|   IBIS model for TI TMS320TCI6457 DSP
[IBIS Ver]   5.0
[Disclaimer]   Please be aware that in the absence of a written agreement
|   Texas Instruments(TI) assumes no liability for:
|   (1) The accuracy of the IBIS models provided to your company
|   (2) The proper functioning of these Models in your design
|   or for any resulting applications
|   (3) Infringement of patents, copyrights or intellectual
|   property rights resulting from your use of these
|   models.
|   TI provides IBIS Models as a service to our customers and
|   therefore reserves the right to limit distribution of the
|   Models.  The information is subject to change without notice.
[File Name]  tms320c6457c.ibs
[File Rev]   1.2
[Date]   March 30, 2011
[Source]   File Originated at Texas Instruments
|   Revision 1.2 -- 30 March 2011 - [R. Lerner]
|   -Updated bshtltcscdvgpbfz ibis model
|   -IBISCHK5 resulted in 0 errors and 37 warnings (listed below)
|   Revision 1.1 -- 2/14/2011
|   cleaned uprevision history
|   -108 Warnings identified
|   Revision 1.0 -- 5/26/2010 [Initial full release]
|   Updated IO buffer models added
|   -BC1840DTHYPDFZ
|   -BC1840ETHYFZ
|   -ICLKRX18G
|   -IC18THYPUFZ
|   -IC18THYPDFZ
|   -IC18THY
|   -IC18GHY
|   -BSHTLTCSCDVGPBFZ
|   the following portions of the model have been updated
|   Driver:
|   a) Impedance   - 45/50/55 ohms impedance
|   b) Slew Rate Operation   - Fast and slow modes of operation
|   c) Voltage Levels   - 1.5/1.8V
|   d) Voltage Nom variation   - 10%/5%
|   Reciever -
|   a) Termination Modes  - Half/Full Termination as well as no termination modes
|   b) Termination Impedance   - 45/50/55 ohms impedance
|   c) Voltage Levels   - 1.5/1.8V
|   d) Voltage Nom variation   - 10%/5%
|   -BI2C18TFZ
|   -BC1850CTHYPUFZ
|   -BC1840ETHYPDFZ
|   -BC1825ETHYPUFZ
|   -BC1825ETHYPDFZ
|   -BQ3350ZTCBTHYPBFZP18
|   -BQ3340ZTCDTHYPBFZP18
|   -BC1850CTHYPDFZ
|   Note: Updated BC1825ETHYPUFZ model missing
|   IBIS Checker updated
|   IBIS Quality Notes added
|   File passes ibischk5.0.3 with 0 errors and 4 warnings.
|   Revision 0.3 -- 1/29/2009
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[Copyright]   Property of Texas Instruments Incorporated.
|   Unauthorized reproduction and/or distribution is strictly
|   prohibited.
|   This product is protected under copyright law and trade
|   secret law as an unpublished work.
|   Created 2008,(C) Copyright 1999-2011,
|   Texas Instruments Incorporated., All Rights Reserved.
|   These commodities are under the U.S.
|   Government distribution license control.As such,they are not
|   to be re-exported without the prior approval of the U.S.
|   Department of Commerce.
[Notes]
|   Some IV curves contain Non monotonic data points.
|   Some reserved pins (RSVxx) are listed as NC, these pins may
|   require either a pull up or pull down resistor to the
|   appropriate rail - refer to your data manual for proper connection
|   IBIS Quality Notes
|   Component TMS320TCI6457: Over all Quality Level 2A
|  IQ
|  IQ  IBISCHK5 V5.0.4
|  IQ
|  IQ  Buffer Model BC1840DTHYPDFZ: IQ Level 2A
|  IQ   -Warning: POWER Clamp, Typical value never becomes zero
|  IQ   -Warning: POWER Clamp, Minimum value never becomes zero
|  IQ   -Warning: POWER Clamp, Maximum value never becomes zero
|  IQ   -Note: Pull down/up min/typ/max data is non-monotonic
|  IQ  Buffer Model ICLKRX18G: IQ Level 2A
|  IQ   -Warning: POWER Clamp, Typical value never becomes zero
|  IQ   -Warning: POWER Clamp, Minimum value never becomes zero
|  IQ   -Warning: POWER Clamp, Maximum value never becomes zero
|  IQ   -Note: Pull down/up min/typ/max data is non-monotonic
|  IQ  Buffer Model IC18THYPUFZ: IQ Level 2A
|  IQ   -Warning: GND Clamp, Typical value never becomes zero
|  IQ   -Warning: GND Clamp, Maximum value never becomes zero
|  IQ   -Note: Pull down/up min/typ/max data is non-monotonic
|  IQ  Buffer Model IC18THYPDFZ: IQ Level 2A
|  IQ   -Warning: POWER Clamp, Typical value never becomes zero
|  IQ   -Warning: POWER Clamp, Minimum value never becomes zero
|  IQ   -Warning: POWER Clamp, Maximum value never becomes zero
|  IQ  Buffer Model BC1850CTHYPUFZ: IQ Level 2A
|  IQ   -Warning: GND Clamp, Typical value never becomes zero
|  IQ   -Warning: GND Clamp, Maximum value never becomes zero
|  IQ   -Note: Pull down/up min/typ/max data is non-monotonic
|  IQ  Buffer Model BC1840ETHYPDFZ: IQ Level 2A
|  IQ   -Warning: POWER Clamp, Typical value never becomes zero
|  IQ   -Warning: POWER Clamp, Minimum value never becomes zero
|  IQ   -Warning: POWER Clamp, Maximum value never becomes zero
|  IQ   -Note: Pull down/up min/typ/max data is non-monotonic
|  IQ  Buffer Model BC1825ETHYPUFZ: IQ Level 2A
|  IQ   -Warning: GND Clamp, Typical value never becomes zero
|  IQ   -Warning: GND Clamp, Maximum value never becomes zero
|  IQ   -Note: Pull down/up min/typ/max data is non-monotonic
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[Component] TMS320C6457
[Manufacturer] Texas Instruments
[Package Model] 6457
[Package]
||Variable   Typ   Min   Max
R_pkg   1.77   0.845   3.51
L_pkg   3.61nH  2.22nH   6.22nH
C_pkg   1.76pF  1.22pF   2.84pF
[Pin]   signal_name   model_name
G6   DDRCLKSEL   IC18GHY
AE19   NMI   BC1850CTHYPDFZ
AF6   ALTCORECLK   IC18THY
AF23   RESETSTATZ   BC1850CTHYPDFZ
AH6   CORECLKP   ICLKRX18G
AH23   RESETZ   IC18THY
AD7   SYSCLKOUT   BC1840ETHYPDFZ
AG22   PORZ   IC18THY
AG7   RIOSGMIICLKP   ICLKRX18G
AG6   RIOSGMIICLKN   ICLKRX18G
AE6   CORECLKSEL   IC18GHY
E6   DDRREFCLKN   ICLKRX18G
D6   DDRREFCLKP   ICLKRX18G
AH7   CORECLKN   ICLKRX18G
C6   ALTDDRCLK   IC18THY
E22   DDRDQS3P   BSHTLTCSCDVGPBFZ
B6   DDRD14   BSHTLTCSCDVGPBFZ
E8   DDRD10   BSHTLTCSCDVGPBFZ
A15   DDRA11   BSHTLTCSCDVGPBFZ
C8   DDRD08   BSHTLTCSCDVGPBFZ
D21   DDRD27   BSHTLTCSCDVGPBFZ
D18   DDRD19   BSHTLTCSCDVGPBFZ
A24   DDRD30   BSHTLTCSCDVGPBFZ
C12   DDRWEZ   BSHTLTCSCDVGPBFZ
C19   DDRDQM2   BSHTLTCSCDVGPBFZ
A27   DDRSLRATE   BC1840ETHYFZ
A21   DDRD24   BSHTLTCSCDVGPBFZ
D11   DDRD03   BSHTLTCSCDVGPBFZ
D7   DDRDQS1N   BSHTLTCSCDVGPBFZ
F17   DDRA00   BSHTLTCSCDVGPBFZ
B21   DDRD25   BSHTLTCSCDVGPBFZ
B17   DDRCLKOUTN1   BSHTLTCSCDVGPBFZ
E17   DDRA01   BSHTLTCSCDVGPBFZ
C16   DDRA06   BSHTLTCSCDVGPBFZ
C22   DDRDQM3   BSHTLTCSCDVGPBFZ
A20   DDRD20   BSHTLTCSCDVGPBFZ
B15   DDRA10   BSHTLTCSCDVGPBFZ
E13   DDRCEZ   BSHTLTCSCDVGPBFZ
C11   DDRD02   BSHTLTCSCDVGPBFZ
C17   DDRA03   BSHTLTCSCDVGPBFZ
D20   DDRD23   BSHTLTCSCDVGPBFZ
D8   DDRD09   BSHTLTCSCDVGPBFZ
D19   DDRDQS2N   BSHTLTCSCDVGPBFZ
A10   DDRD04   BSHTLTCSCDVGPBFZ
C15   DDRA09   BSHTLTCSCDVGPBFZ
D16   DDRA05   BSHTLTCSCDVGPBFZ
B16   DDRA07   BSHTLTCSCDVGPBFZ
E10   DDRDQS0P   BSHTLTCSCDVGPBFZ
B12   DDRD01   BSHTLTCSCDVGPBFZ
B9   DDRRCVENOUT0   BSHTLTCSCDVGPBFZ
F20   DDRRCVENOUT1   BSHTLTCSCDVGPBFZ
D12   DDRRASZ   BSHTLTCSCDVGPBFZ
E16   DDRA04   BSHTLTCSCDVGPBFZ
E15   DDRODT   BSHTLTCSCDVGPBFZ
C18   DDRD18   BSHTLTCSCDVGPBFZ
D13   DDRCKE   BSHTLTCSCDVGPBFZ
A18   DDRD17   BSHTLTCSCDVGPBFZ
E7   DDRDQS1P   BSHTLTCSCDVGPBFZ
B10   DDRD05   BSHTLTCSCDVGPBFZ
B14   DDRA13   BSHTLTCSCDVGPBFZ
D14   DDRBA1   BSHTLTCSCDVGPBFZ
A14   DDRA12   BSHTLTCSCDVGPBFZ
B23   DDRD29   BSHTLTCSCDVGPBFZ
E19   DDRDQS2P   BSHTLTCSCDVGPBFZ
E20   DDRRCVENIN1   BSHTLTCSCDVGPBFZ
E12   DDRCASZ   BSHTLTCSCDVGPBFZ
B20   DDRD21   BSHTLTCSCDVGPBFZ
B13   DDRCLKOUTN0   BSHTLTCSCDVGPBFZ
A6   DDRD15   BSHTLTCSCDVGPBFZ
C7   DDRDQM1   BSHTLTCSCDVGPBFZ
A9   DDRRCVENIN0   BSHTLTCSCDVGPBFZ
C21   DDRD26   BSHTLTCSCDVGPBFZ
D17   DDRA02   BSHTLTCSCDVGPBFZ
F8   DDRD11   BSHTLTCSCDVGPBFZ
A17   DDRCLKOUTP1   BSHTLTCSCDVGPBFZ
B18   DDRD16   BSHTLTCSCDVGPBFZ
D15   DDRA08   BSHTLTCSCDVGPBFZ
E14   DDRBA2   BSHTLTCSCDVGPBFZ
B24   DDRD31   BSHTLTCSCDVGPBFZ
A23   DDRD28   BSHTLTCSCDVGPBFZ
D22   DDRDQS3N   BSHTLTCSCDVGPBFZ
B7   DDRD12   BSHTLTCSCDVGPBFZ
A13   DDRCLKOUTP0   BSHTLTCSCDVGPBFZ
D10   DDRDQS0N   BSHTLTCSCDVGPBFZ
D9   DDRD07   BSHTLTCSCDVGPBFZ
C10   DDRDQM0   BSHTLTCSCDVGPBFZ
C20   DDRD22   BSHTLTCSCDVGPBFZ
C9   DDRD06   BSHTLTCSCDVGPBFZ
C14   DDRBA0   BSHTLTCSCDVGPBFZ
A7   DDRD13   BSHTLTCSCDVGPBFZ
A12   DDRD00   BSHTLTCSCDVGPBFZ
P25   AEA16   BQ3350ZTCBTHYPBFZP18
AD26   AED12   BQ3350ZTCBTHYPBFZP18
AF24   AED03   BQ3350ZTCBTHYPBFZP18
N26   AEA07   BQ3350ZTCBTHYPBFZP18
U25   AEA00   BQ3350ZTCBTHYPBFZP18
V25   ABA0   BQ3350ZTCBTHYPBFZP18
F27   AED52   BQ3350ZTCBTHYPBFZP18
T25   AEA11   BQ3350ZTCBTHYPBFZP18
G26   AED50   BQ3350ZTCBTHYPBFZP18
AB25   AED26   BQ3350ZTCBTHYPBFZP18
H26   AED43   BQ3350ZTCBTHYPBFZP18
Y27   AED27   BQ3350ZTCBTHYPBFZP18
AC24   AED00   BQ3350ZTCBTHYPBFZP18
C28   AED41   BQ3350ZTCBTHYPBFZP18
J24   AED47   BQ3350ZTCBTHYPBFZP18
R26   AEA13   BQ3350ZTCBTHYPBFZP18
G27   AED48   BQ3350ZTCBTHYPBFZP18
AF28   AED30   BQ3350ZTCBTHYPBFZP18
B27   AED51   BQ3350ZTCBTHYPBFZP18
W27   ABE02Z   BQ3350ZTCBTHYPBFZP18
D25   AED57   BQ3350ZTCBTHYPBFZP18
D28   AED39   BQ3350ZTCBTHYPBFZP18
K25   AED46   BQ3350ZTCBTHYPBFZP18
AA24   ASDWEZ   BQ3350ZTCBTHYPBFZP18
L24   AED33   BQ3350ZTCBTHYPBFZP18
AE28   AED19   BQ3350ZTCBTHYPBFZP18
U28   AEA05   BQ3350ZTCBTHYPBFZP18
AE25   AOE   BQ3350ZTCBTHYPBFZP18
AG25   AED14   BQ3350ZTCBTHYPBFZP18
AB26   AED28   BQ3350ZTCBTHYPBFZP18
AA27   AED22   BQ3350ZTCBTHYPBFZP18
AF25   AED09   BQ3350ZTCBTHYPBFZP18
V26   ACE5Z   BQ3350ZTCBTHYPBFZP18
G25   AED36   BQ3350ZTCBTHYPBFZP18
R25   AADS   BQ3350ZTCBTHYPBFZP18
Y24   ABE01Z   BQ3350ZTCBTHYPBFZP18
AA25   AED23   BQ3350ZTCBTHYPBFZP18
T26   AEA02   BQ3350ZTCBTHYPBFZP18
N25   AHOLDAZ   BQ3350ZTCBTHYPBFZP18
J25   AED45   BQ3350ZTCBTHYPBFZP18
AC25   AED11   BQ3350ZTCBTHYPBFZP18
AB24   AED24   BQ3350ZTCBTHYPBFZP18
M26   AEA09   BQ3350ZTCBTHYPBFZP18
Y28   ABE03Z   BQ3350ZTCBTHYPBFZP18
G28   AED35   BQ3350ZTCBTHYPBFZP18
AE24   AED01   BQ3350ZTCBTHYPBFZP18
K28   AARDY   BQ3350ZTCBTHYPBFZP18
L28   ABE05Z   BQ3350ZTCBTHYPBFZP18
M24   AEA17   BQ3350ZTCBTHYPBFZP18
AC26   AED08   BQ3350ZTCBTHYPBFZP18
D27   AED58   BQ3350ZTCBTHYPBFZP18
W26   ACE2Z   BQ3350ZTCBTHYPBFZP18
AA28   AED29   BQ3350ZTCBTHYPBFZP18
N24   AEA10   BQ3350ZTCBTHYPBFZP18
E26   AED59   BQ3350ZTCBTHYPBFZP18
AE27   AED15   BQ3350ZTCBTHYPBFZP18
AF27   AED18   BQ3350ZTCBTHYPBFZP18
V24   ABA1   BQ3350ZTCBTHYPBFZP18
B26   AED49   BQ3350ZTCBTHYPBFZP18
C26   AED61   BQ3350ZTCBTHYPBFZP18
T28   AEA06   BQ3350ZTCBTHYPBFZP18
H24   AED55   BQ3350ZTCBTHYPBFZP18
AG27   AED20   BQ3350ZTCBTHYPBFZP18
U27   ACE4Z   BQ3350ZTCBTHYPBFZP18
J28   AED40   BQ3350ZTCBTHYPBFZP18
AC27   AED13   BQ3350ZTCBTHYPBFZP18
W28   ABE07Z   BQ3350ZTCBTHYPBFZP18
D26   AED53   BQ3350ZTCBTHYPBFZP18
T27   AEA03   BQ3350ZTCBTHYPBFZP18
AD27   AED04   BQ3350ZTCBTHYPBFZP18
AH26   AED06   BQ3350ZTCBTHYPBFZP18
N28   AECLKIN   BQ3350ZTCBTHYPBFZP18
Y25   ABE00Z   BQ3350ZTCBTHYPBFZP18
J26   AED44   BQ3350ZTCBTHYPBFZP18
A26   AED62   BQ3350ZTCBTHYPBFZP18
C27   AED60   BQ3350ZTCBTHYPBFZP18
H25   AED54   BQ3350ZTCBTHYPBFZP18
AF26   AED16   BQ3350ZTCBTHYPBFZP18
M25   AEA18   BQ3350ZTCBTHYPBFZP18
L27   ABE04Z   BQ3350ZTCBTHYPBFZP18
AE26   AED10   BQ3350ZTCBTHYPBFZP18
G24   AED63   BQ3350ZTCBTHYPBFZP18
K27   AED34   BQ3350ZTCBTHYPBFZP18
L26   ABUSREQ0   BQ3350ZTCBTHYPBFZP18
K24   AED38   BQ3350ZTCBTHYPBFZP18
U26   AEA01   BQ3350ZTCBTHYPBFZP18
Y26   AED31   BQ3350ZTCBTHYPBFZP18
W25   ACE3Z   BQ3350ZTCBTHYPBFZP18
P24   AEA19   BQ3350ZTCBTHYPBFZP18
AD28   AED17   BQ3350ZTCBTHYPBFZP18
F26   AED56   BQ3350ZTCBTHYPBFZP18
W24   ARNW   BQ3350ZTCBTHYPBFZP18
T24   AEA14   BQ3350ZTCBTHYPBFZP18
R24   AEA08   BQ3350ZTCBTHYPBFZP18
R27   AEA04   BQ3350ZTCBTHYPBFZP18
F28   AED37   BQ3350ZTCBTHYPBFZP18
P26   AEA15   BQ3350ZTCBTHYPBFZP18
J27   AED42   BQ3350ZTCBTHYPBFZP18
K26   AED32   BQ3350ZTCBTHYPBFZP18
N27   AEA12   BQ3350ZTCBTHYPBFZP18
AG26   AED02   BQ3350ZTCBTHYPBFZP18
AH25   AED05   BQ3350ZTCBTHYPBFZP18
AC28   AED21   BQ3350ZTCBTHYPBFZP18
V28   AECLKOUT   BQ3340ZTCDTHYPBFZP18
L25   ABE06Z   BQ3350ZTCBTHYPBFZP18
R28   AHOLDZ   BQ3350ZTCBTHYPBFZP18
AA26   AED25   BQ3350ZTCBTHYPBFZP18
AD25   AED07   BQ3350ZTCBTHYPBFZP18
AE4   EMU03   BC1825ETHYPUFZ
AH5   EMU02   BC1825ETHYPUFZ
AD5   EMU00   BC1825ETHYPUFZ
AD1   EMU15   BC1825ETHYPUFZ
AE3   EMU10   BC1825ETHYPUFZ
AG4   EMU05   BC1825ETHYPUFZ
AF2   EMU11   BC1825ETHYPUFZ
Y2   TMS   IC18THYPUFZ
AA1   EMU17   BC1825ETHYPUFZ
AE1   EMU12   BC1825ETHYPUFZ
AG2   EMU07   BC1825ETHYPUFZ
AB1   TDI   IC18THYPUFZ
AF3   EMU13   BC1825ETHYPUFZ
AF4   EMU06   BC1825ETHYPUFZ
AC1   EMU14   BC1825ETHYPUFZ
AD3   EMU16   BC1825ETHYPUFZ
AH3   TCK   IC18THYPUFZ
AC2   EMU18   BC1825ETHYPUFZ
AE5   EMU01   BC1825ETHYPUFZ
AH4   EMU04   BC1825ETHYPUFZ
AE2   TRSTZ   IC18THYPDFZ
AG3   EMU08   BC1825ETHYPUFZ
AF1   TDO   BC1840ETHYFZ
AD4   EMU09   BC1825ETHYPUFZ
D24   GP12   BC1825ETHYPDFZ
B25   GP08   BC1825ETHYPDFZ
C5   GP06   BC1825ETHYPDFZ
B5   GP04   BC1825ETHYPDFZ
F5   GP07   BC1825ETHYPDFZ
C25   GP11   BC1825ETHYPDFZ
B4   GP03   BC1825ETHYPDFZ
D5   GP02   BC1825ETHYPDFZ
A5   GP00   BC1825ETHYPUFZ
E5   GP01   BC1825ETHYPDFZ
A25   GP10   BC1825ETHYPDFZ
F6   GP05   BC1825ETHYPDFZ
C24   GP09   BC1825ETHYPDFZ
D23   GP14   BC1825ETHYPDFZ
F23   GP15   BC1825ETHYPDFZ
C23   GP13   BC1825ETHYPDFZ
R1   HD17   BQ3350ZTCBTHYPBFZP18
W1   HD11   BQ3350ZTCBTHYPBFZP18
P3   HD31   BQ3350ZTCBTHYPBFZP18
V1   HD22   BQ3350ZTCBTHYPBFZP18
T3   HD09   BQ3350ZTCBTHYPBFZP18
L2   HDS1Z   BQ3350ZTCBTHYPBFZP18
M1   HD24   BQ3350ZTCBTHYPBFZP18
W2   HD00   BQ3350ZTCBTHYPBFZP18
L6   HCNTL0   BQ3350ZTCBTHYPBFZP18
N4   HD12   BQ3350ZTCBTHYPBFZP18
U4   HD05   BQ3350ZTCBTHYPBFZP18
R6   HD04   BQ3350ZTCBTHYPBFZP18
N3   HD16   BQ3350ZTCBTHYPBFZP18
N5   HD08   BQ3350ZTCBTHYPBFZP18
R5   HD10   BQ3350ZTCBTHYPBFZP18
P4   HD14   BQ3350ZTCBTHYPBFZP18
U5   HD27   BQ3350ZTCBTHYPBFZP18
M6   HRDYZ   BQ3350ZTCBTHYPBFZP18
N1   HD26   BQ3350ZTCBTHYPBFZP18
K5   HRWZ   BQ3350ZTCBTHYPBFZP18
L3   HHWIL   BQ3350ZTCBTHYPBFZP18
N2   HD20   BQ3350ZTCBTHYPBFZP18
U1   HD21   BQ3350ZTCBTHYPBFZP18
T1   HD19   BQ3350ZTCBTHYPBFZP18
P5   HD02   BQ3350ZTCBTHYPBFZP18
T2   HD15   BQ3350ZTCBTHYPBFZP18
M3   HCSZ   BQ3350ZTCBTHYPBFZP18
N6   HD30   BQ3350ZTCBTHYPBFZP18
T5   HD29   BQ3350ZTCBTHYPBFZP18
M5   HCNTL1   BQ3350ZTCBTHYPBFZP18
U6   HD23   BQ3350ZTCBTHYPBFZP18
K6   HD01   BQ3350ZTCBTHYPBFZP18
L4   HINTZ   BQ3350ZTCBTHYPBFZP18
P2   HD18   BQ3350ZTCBTHYPBFZP18
T4   HD03   BQ3350ZTCBTHYPBFZP18
R4   HD07   BQ3350ZTCBTHYPBFZP18
P6   HD28   BQ3350ZTCBTHYPBFZP18
U2   HD13   BQ3350ZTCBTHYPBFZP18
L5   HDS2Z   BQ3350ZTCBTHYPBFZP18
M4   HASZ   BQ3350ZTCBTHYPBFZP18
T6   HD06   BQ3350ZTCBTHYPBFZP18
V2   HD25   BQ3350ZTCBTHYPBFZP18
F24   SCL   BI2C18TFZ
E24   SDA   BI2C18TFZ
Y6   DR0   IC18THYPDFZ
AA4   CLKS0   IC18THYPDFZ
V4   FSR0   BC1840DTHYPDFZ
W4   FSX0   BC1840DTHYPDFZ
Y5   CLKR0   BC1840DTHYPDFZ
AB3   CLKX0   BC1840DTHYPDFZ
W6   DX0   BC1840DTHYPDFZ
AA3   CLKX1   BC1840DTHYPDFZ
Y3   DX1   BC1840DTHYPDFZ
W3   DR1   IC18THYPDFZ
V5   FSR1   BC1840DTHYPDFZ
Y1   CLKS1   IC18THYPDFZ
W5   FSX1   BC1840DTHYPDFZ
Y4   CLKR1   BC1840DTHYPDFZ
AH19   MDIO   BC1850CTHYPUFZ
AH18   MDCLK   BC1850CTHYPDFZ
AG19   TINP1L   IC18THYPDFZ
AF19   TOUT1L   BC1825ETHYPDFZ
AG20   TOUT0L   BC1825ETHYPDFZ
AH20   TINP0L   IC18THYPDFZ
H3   UXDATA3   BQ3350ZTCBTHYPBFZP18
H2   URADDR0   BQ3350ZTCBTHYPBFZP18
K1   URADDR4   BQ3350ZTCBTHYPBFZP18
J5   UXADDR1   BQ3350ZTCBTHYPBFZP18
J1   URADDR2   BQ3350ZTCBTHYPBFZP18
F2   URDATA6   BQ3350ZTCBTHYPBFZP18
K2   URADDR3   BQ3350ZTCBTHYPBFZP18
H5   UXADDR3   BQ3350ZTCBTHYPBFZP18
G3   UXDATA2   BQ3350ZTCBTHYPBFZP18
C4   UXDATA5   BQ3350ZTCBTHYPBFZP18
F1   URDATA5   BQ3350ZTCBTHYPBFZP18
E1   URDATA3   BQ3350ZTCBTHYPBFZP18
C3   UXCLAV   BQ3350ZTCBTHYPBFZP18
C1   URCLK   BQ3350ZTCBTHYPBFZP18
K3   UXADDR2   BQ3350ZTCBTHYPBFZP18
F3   UXDATA7   BQ3350ZTCBTHYPBFZP18
E3   UXDATA0   BQ3350ZTCBTHYPBFZP18
B3   UXENBZ   BQ3350ZTCBTHYPBFZP18
G2   URSOC   BQ3350ZTCBTHYPBFZP18
E4   UXDATA6   BQ3350ZTCBTHYPBFZP18
A3   UXDATA4   BQ3350ZTCBTHYPBFZP18
D2   URDATA2   BQ3350ZTCBTHYPBFZP18
D1   URDATA1   BQ3350ZTCBTHYPBFZP18
A4   UXCLK   BQ3350ZTCBTHYPBFZP18
G4   UXSOC   BQ3350ZTCBTHYPBFZP18
C2   URDATA0   BQ3350ZTCBTHYPBFZP18
E2   URDATA4   BQ3350ZTCBTHYPBFZP18
K4   URENBZ   BQ3350ZTCBTHYPBFZP18
H4   UXADDR0   BQ3350ZTCBTHYPBFZP18
J3   URADDR1   BQ3350ZTCBTHYPBFZP18
G1   URDATA7   BQ3350ZTCBTHYPBFZP18
F4   UXDATA1   BQ3350ZTCBTHYPBFZP18
B2   URCLAV   BQ3350ZTCBTHYPBFZP18
J4   UXADDR4   BQ3350ZTCBTHYPBFZP18
AC5   PLLV1   Power
F7   PLLV2   Power
K10   CVdd   Power
K12   CVdd   Power
K14   CVdd   Power
K16   CVdd   Power
K18   CVdd   Power
L11   CVdd   Power
L13   CVdd   Power
L15   CVdd   Power
L17   CVdd   Power
L19   CVdd   Power
M10   CVdd   Power
M12   CVdd   Power
M14   CVdd   Power
M16   CVdd   Power
M18   CVdd   Power
N11   CVdd   Power
N13   CVdd   Power
N15   CVdd   Power
N17   CVdd   Power
N19   CVdd   Power
P10   CVdd   Power
P12   CVdd   Power
P14   CVdd   Power
P16   CVdd   Power
P18   CVdd   Power
R11   CVdd   Power
R13   CVdd   Power
R15   CVdd   Power
R17   CVdd   Power
R19   CVdd   Power
T12   CVdd   Power
T14   CVdd   Power
T16   CVdd   Power
T18   CVdd   Power
U11   CVdd   Power
U15   CVdd   Power
U17   CVdd   Power
V10   CVdd   Power
V16   CVdd   Power
V18   CVdd   Power
W17   CVdd   Power
W19   CVdd   Power
A16   PVT18   Power
U19   CVDDMON   Power
U22   DVDD33MON   Power
G23   DVDD18MON   Power
AE10   VDDR18   Power
AE16   VDDR18   Power
AC10   SGR_VDDA11   Power
AC12   SGR_VDDA11   Power
AC14   SGR_VDDA11   Power
AC16   SGR_VDDA11   Power
U13   SGR_VDDD11   Power
V12   SGR_VDDD11   Power
V14   SGR_VDDD11   Power
W11   SGR_VDDD11   Power
W13   SGR_VDDD11   Power
W15   SGR_VDDD11   Power
AD9   SGR_VDDT11   Power
AD11   SGR_VDDT11   Power
AD13   SGR_VDDT11   Power
AD15   SGR_VDDT11   Power
AD17   SGR_VDDT11   Power
AF9   SGR_VDDT11   Power
AF15   SGR_VDDT11   Power
AG11   SGR_VDDT11   Power
AH17   SGR_VDDT11   Power
AA6   DVDD18   Power
AB18   DVDD18   Power
AB20   DVDD18   Power
AB7   DVDD18   Power
AC19   DVDD18   Power
AC21   DVDD18   Power
AC3   DVDD18   Power
AC8   DVDD18   Power
AD18   DVDD18   Power
AD22   DVDD18   Power
AF18   DVDD18   Power
AG5   DVDD18   Power
AH1   DVDD18   Power
B11   DVDD18   Power
B19   DVDD18   Power
B22   DVDD18   Power
B8   DVDD18   Power
E11   DVDD18   Power
E21   DVDD18   Power
E23   DVDD18   Power
E9   DVDD18   Power
F10   DVDD18   Power
F12   DVDD18   Power
F14   DVDD18   Power
F16   DVDD18   Power
F18   DVDD18   Power
G11   DVDD18   Power
G13   DVDD18   Power
G15   DVDD18   Power
G17   DVDD18   Power
G19   DVDD18   Power
G21   DVDD18   Power
G7   DVDD18   Power
G9   DVDD18   Power
J7   DVDD18   Power
V6   DVDD18   Power
Y7   DVDD18   Power
A1   DVDD33   Power
A28   DVDD33   Power
AA23   DVDD33   Power
AB22   DVDD33   Power
AB28   DVDD33   Power
AC23   DVDD33   Power
AD24   DVDD33   Power
AH24   DVDD33   Power
AH28   DVDD33   Power
D3   DVDD33   Power
E25   DVDD33   Power
E27   DVDD33   Power
H1   DVDD33   Power
H22   DVDD33   Power
H27   DVDD33   Power
J23   DVDD33   Power
K22   DVDD33   Power
L1   DVDD33   Power
L23   DVDD33   Power
L7   DVDD33   Power
M22   DVDD33   Power
M27   DVDD33   Power
N23   DVDD33   Power
N7   DVDD33   Power
P1   DVDD33   Power
P22   DVDD33   Power
P27   DVDD33   Power
R23   DVDD33   Power
R3   DVDD33   Power
R7   DVDD33   Power
T22   DVDD33   Power
U7   DVDD33   Power
V22   DVDD33   Power
V3   DVDD33   Power
W23   DVDD33   Power
Y22   DVDD33   Power
A11   Vss   GND
A19   Vss   GND
A2   Vss   GND
A22   Vss   GND
A8   Vss   GND
AA2   Vss   GND
AA22   Vss   GND
AA7   Vss   GND
AB10   Vss   GND
AB11   Vss   GND
AB12   Vss   GND
AB13   Vss   GND
AB14   Vss   GND
AB15   Vss   GND
AB16   Vss   GND
AB17   Vss   GND
AB19   Vss   GND
AB21   Vss   GND
AB23   Vss   GND
AB27   Vss   GND
AB6   Vss   GND
AB8   Vss   GND
AB9   Vss   GND
AC11   Vss   GND
AC13   Vss   GND
AC15   Vss   GND
AC17   Vss   GND
AC18   Vss   GND
AC20   Vss   GND
AC22   Vss   GND
AC9   Vss   GND
AD10   Vss   GND
AD12   Vss   GND
AD14   Vss   GND
AD16   Vss   GND
AD19   Vss   GND
AD2   Vss   GND
AD23   Vss   GND
AD8   Vss   GND
AE11   Vss   GND
AE14   Vss   GND
AE15   Vss   GND
AE17   Vss   GND
AE18   Vss   GND
AF5   Vss   GND
AF8   Vss   GND
AG1   Vss   GND
AG10   Vss   GND
AG12   Vss   GND
AG15   Vss   GND
AG17   Vss   GND
AG18   Vss   GND
AG24   Vss   GND
AG28   Vss   GND
AH11   Vss   GND
AH16   Vss   GND
AH2   Vss   GND
AH27   Vss   GND
AH8   Vss   GND
B1   Vss   GND
B28   Vss   GND
D4   Vss   GND
E18   Vss   GND
E28   Vss   GND
F11   Vss   GND
F13   Vss   GND
F15   Vss   GND
F19   Vss   GND
F21   Vss   GND
F22   Vss   GND
F25   Vss   GND
F9   Vss   GND
G10   Vss   GND
G12   Vss   GND
G14   Vss   GND
G16   Vss   GND
G18   Vss   GND
G20   Vss   GND
G22   Vss   GND
G8   Vss   GND
H23   Vss   GND
H28   Vss   GND
H7   Vss   GND
J2   Vss   GND
J22   Vss   GND
K11   Vss   GND
K13   Vss   GND
K15   Vss   GND
K17   Vss   GND
K19   Vss   GND
K23   Vss   GND
K7   Vss   GND
L10   Vss   GND
L12   Vss   GND
L14   Vss   GND
L16   Vss   GND
L18   Vss   GND
L22   Vss   GND
M11   Vss   GND
M13   Vss   GND
M15   Vss   GND
M17   Vss   GND
M19   Vss   GND
M2   Vss   GND
M23   Vss   GND
M28   Vss   GND
M7   Vss   GND
N10   Vss   GND
N12   Vss   GND
N14   Vss   GND
N16   Vss   GND
N18   Vss   GND
N22   Vss   GND
P11   Vss   GND
P13   Vss   GND
P15   Vss   GND
P17   Vss   GND
P19   Vss   GND
P23   Vss   GND
P28   Vss   GND
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|   Component BSHTLTCSCDVGPBFZ
[Model Selector] BSHTLTCSCDVGPBFZ
|   -The designation "SR" refers to Slew Rate
|   -The designation 1p8" refers to 1.8 where "p" refers to "point"
|   -The designation "NOSR" refers to No Slew Rate
|   -The designation "10PER" refers to 10 percent
|   -The designation "NOTERM" refers to no thevenin termination
|   -The designation "HALFTERM" refers to half thevenin termination
|   -The designation "FULLTERM" refers to full thevenin termination
NOSR0_10PER_45OHM_1P8  TX MODE,1.8V +/- 10PERCENT,45OHM,FAST SLEWRATE (SR0=0)
|NOSR0_10PER_45OHM_1P8;
SR0_10PER_45OHM_1P8  TX MODE,1.8V +/- 10PERCENT,45OHM,SLOW SLEWRATE (SR0=1)
|SR0_10PER_45OHM_1P8;
NOSR0_5PER_45OHM_1P8  TX MODE,1.8V +/- 5PERCENT,45OHM,FAST SLEWRATE (SR0=0)
|NOSR0_5PER_45OHM_1P8;
SR0_5PER_45OHM_1P8  TX MODE,1.8V +/- 5PERCENT,45OHM,SLOW SLEWRATE (SR0=1)
|SR0_5PER_45OHM_1P8;
NOSR0_10PER_50OHM_1P8  TX MODE,1.8V +/- 10PERCENT,50OHM,FAST SLEWRATE (SR0=0)
|NOSR0_10PER_50OHM_1P8;
SR0_10PER_50OHM_1P8  TX MODE,1.8V +/- 10PERCENT,50OHM,SLOW SLEWRATE (SR0=1)
|SR0_10PER_50OHM_1P8;
NOSR0_5PER_50OHM_1P8  TX MODE,1.8V +/- 5PERCENT,50OHM,FAST SLEWRATE (SR0=0)
|NOSR0_5PER_50OHM_1P8;
SR0_5PER_50OHM_1P8  TX MODE,1.8V +/- 5PERCENT,50OHM,SLOW SLEWRATE (SR0=1)
|SR0_5PER_50OHM_1P8;
NOSR0_10PER_55OHM_1P8  TX MODE,1.8V +/- 10PERCENT,55OHM,FAST SLEWRATE (SR0=0)
|NOSR0_10PER_55OHM_1P8;
SR0_10PER_55OHM_1P8  TX MODE,1.8V +/- 10PERCENT,55OHM,SLOW SLEWRATE (SR0=1)
|SR0_10PER_55OHM_1P8;
NOSR0_5PER_55OHM_1P8  TX MODE,1.8V +/- 5PERCENT,55OHM,FAST SLEWRATE (SR0=0)
|NOSR0_5PER_55OHM_1P8;
SR0_5PER_55OHM_1P8  TX MODE,1.8V +/- 5PERCENT,55OHM,SLOW SLEWRATE (SR0=1)
|SR0_5PER_55OHM_1P8;
NOSR0_10PER_30OHM_1P8  TX MODE,1.8V +/- 10PERCENT,30OHM,FAST SLEWRATE (SR0=0)
|NOSR0_10PER_30OHM_1P8;
SR0_10PER_30OHM_1P8  TX MODE,1.8V +/- 10PERCENT,30OHM,SLOW SLEWRATE (SR0=1)
|SR0_10PER_30OHM_1P8;
NOSR0_5PER_30OHM_1P8  TX MODE,1.8V +/- 5PERCENT,30OHM,FAST SLEWRATE (SR0=0)
|NOSR0_5PER_30OHM_1P8;
SR0_5PER_30OHM_1P8  TX MODE,1.8V +/- 5PERCENT,30OHM,SLOW SLEWRATE (SR0=1)
|SR0_5PER_30OHM_1P8;
45OHM_10PER_HALFTERM_1P8  RX MODE,1.8V +/- 10PERCENT,90OHM ON DIE TERMINATION
|45OHM_10PER_HALFTERM_1P8;
45OHM_10PER_NOTERM_1P8  RX MODE,1.8V +/- 10PERCENT,WITHOUT TERMINATION
|45OHM_10PER_NOTERM_1P8;
45OHM_10PER_FULLTERM_1P8  RX MODE,1.8V +/- 10PERCENT,45OHM ON DIE TERMINATION
|45OHM_10PER_FULLTERM_1P8;
45OHM_5PER_HALFTERM_1P8  RX MODE,1.8V +/- 5PERCENT,90OHM ON DIE TERMINATION
|45OHM_5PER_HALFTERM_1P8;
45OHM_5PER_NOTERM_1P8  RX MODE,1.8V +/- 5PERCENT,WITHOUT TERMINATION
|45OHM_5PER_NOTERM_1P8;
45OHM_5PER_FULLTERM_1P8  RX MODE,1.8V +/- 5PERCENT,45OHM ON DIE TERMINATION
|45OHM_5PER_FULLTERM_1P8;
50OHM_10PER_HALFTERM_1P8  RX MODE,1.8V +/- 10PERCENT,100OHM ON DIE TERMINATION
|50OHM_10PER_HALFTERM_1P8;
50OHM_10PER_NOTERM_1P8  RX MODE,1.8V +/- 10PERCENT,WITHOUT TERMINATION
|50OHM_10PER_NOTERM_1P8;
50OHM_10PER_FULLTERM_1P8  RX MODE,1.8V +/- 10PERCENT,50OHM ON DIE TERMINATION
|50OHM_10PER_FULLTERM_1P8;
50OHM_5PER_HALFTERM_1P8  RX MODE,1.8V +/- 5PERCENT,100OHM ON DIE TERMINATION
|50OHM_5PER_HALFTERM_1P8;
50OHM_5PER_NOTERM_1P8  RX MODE,1.8V +/- 5PERCENT,WITHOUT TERMINATION
|50OHM_5PER_NOTERM_1P8;
50OHM_5PER_FULLTERM_1P8  RX MODE,1.8V +/- 5PERCENT,50OHM ON DIE TERMINATION
|50OHM_5PER_FULLTERM_1P8;
55OHM_10PER_HALFTERM_1P8  RX MODE,1.8V +/- 10PERCENT,110OHM ON DIE TERMINATION
|55OHM_10PER_HALFTERM_1P8;
55OHM_10PER_NOTERM_1P8  RX MODE,1.8V +/- 10PERCENT,WITHOUT TERMINATION
|55OHM_10PER_NOTERM_1P8;
55OHM_10PER_FULLTERM_1P8  RX MODE,1.8V +/- 10PERCENT,55OHM ON DIE TERMINATION
|55OHM_10PER_FULLTERM_1P8;
55OHM_5PER_HALFTERM_1P8  RX MODE,1.8V +/- 5PERCENT,110OHM ON DIE TERMINATION
|55OHM_5PER_HALFTERM_1P8;
55OHM_5PER_NOTERM_1P8  RX MODE,1.8V +/- 5PERCENT,WITHOUT TERMINATION
|55OHM_5PER_NOTERM_1P8;
55OHM_5PER_FULLTERM_1P8  RX MODE,1.8V +/- 5PERCENT,55OHM ON DIE TERMINATION
|55OHM_5PER_FULLTERM_1P8;
30OHM_10PER_HALFTERM_1P8  RX MODE,1.8V +/- 10PERCENT,60OHM ON DIE TERMINATION
|30OHM_10PER_HALFTERM_1P8;
30OHM_10PER_NOTERM_1P8  RX MODE,1.8V +/- 10PERCENT,WITHOUT TERMINATION
|30OHM_10PER_NOTERM_1P8;
30OHM_10PER_FULLTERM_1P8  RX MODE,1.8V +/- 10PERCENT,30OHM ON DIE TERMINATION
|30OHM_10PER_FULLTERM_1P8;
30OHM_5PER_HALFTERM_1P8  RX MODE,1.8V +/- 5PERCENT,60OHM ON DIE TERMINATION
|30OHM_5PER_HALFTERM_1P8;
30OHM_5PER_NOTERM_1P8  RX MODE,1.8V +/- 5PERCENT,WITHOUT TERMINATION
|30OHM_5PER_NOTERM_1P8;
30OHM_5PER_FULLTERM_1P8  RX MODE,1.8V +/- 5PERCENT,30OHM ON DIE TERMINATION
|30OHM_5PER_FULLTERM_1P8;
[Model Selector] BC1850CTHYPDFZ
BC1850CTHYPDFZ_PD_1P8  Cell operated at 1.8(nom) PULLDOWN_ON
BC1850CTHYPDFZ_PDZ_1P8  Cell operated at 1.8(nom) PULLDOWN_OFF
|   Package Model Definition
[Define Package Model]  6457
[Manufacturer]   Texas Instruments Incorporated
[OEM]   Texas Instruments Incorporated
[Description]   6457 pkg with all signals except SERDES
[Number Of Pins]   344
||added 17Apr09
[Pin Numbers]
G6   |   1   DDRCLKSEL
AE19  |   2   NMI
AF6   |   3   ALTCORECLK
AD6   |   4   RSV24
AF23  |   5   RESETSTATZ
AH6   |   6   CORECLKP
AH23  |   7   RESETZ
G5   |   8   RSV25
AD7   |   9   SYSCLKOUT
AG22  |   10   PORZ
AG7   |   11   RIOSGMIICLKP
AG6   |   12   RIOSGMIICLKN
AE6   |   13   CORECLKSEL
E6   |   14   DDRREFCLKN
D6   |   15   DDRREFCLKP
AH7   |   16   CORECLKN
C6   |   17   ALTDDRCLK
E22   |   18   DDRDQS3P
B6   |   19   DDRD14
E8   |   20   DDRD10
A15   |   21   DDRA11
C8   |   22   DDRD08
D21   |   23   DDRD27
D18   |   24   DDRD19
A24   |   25   DDRD30
C12   |   26   DDRWEZ
C19   |   27   DDRDQM2
A27   |   28   DDRSLRATE
A21   |   29   DDRD24
D11   |   30   DDRD03
D7   |   31   DDRDQS1N
F17   |   32   DDRA00
B21   |   33   DDRD25
B17   |   34   DDRCLKOUTN1
E17   |   35   DDRA01
C16   |   36   DDRA06
C22   |   37   DDRDQM3
A20   |   38   DDRD20
B15   |   39   DDRA10
E13   |   40   DDRCEZ
C11   |   41   DDRD02
C17   |   42   DDRA03
D20   |   43   DDRD23
D8   |   44   DDRD09
D19   |   45   DDRDQS2N
A10   |   46   DDRD04
C15   |   47   DDRA09
D16   |   48   DDRA05
B16   |   49   DDRA07
E10   |   50   DDRDQS0P
B12   |   51   DDRD01
B9   |   52   DDRRCVENOUT0
F20   |   53   DDRRCVENOUT1
D12   |   54   DDRRASZ
E16   |   55   DDRA04
E15   |   56   DDRODT
C18   |   57   DDRD18
D13   |   58   DDRCKE
A18   |   59   DDRD17
E7   |   60   DDRDQS1P
B10   |   61   DDRD05
B14   |   62   DDRA13
D14   |   63   DDRBA1
A14   |   64   DDRA12
B23   |   65   DDRD29
E19   |   66   DDRDQS2P
E20   |   67   DDRRCVENIN1
E12   |   68   DDRCASZ
B20   |   69   DDRD21
B13   |   70   DDRCLKOUTN0
A6   |   71   DDRD15
C7   |   72   DDRDQM1
A9   |   73   DDRRCVENIN0
C21   |   74   DDRD26
D17   |   75   DDRA02
F8   |   76   DDRD11
A17   |   77   DDRCLKOUTP1
B18   |   78   DDRD16
D15   |   79   DDRA08
E14   |   80   DDRBA2
B24   |   81   DDRD31
A23   |   82   DDRD28
D22   |   83   DDRDQS3N
B7   |   84   DDRD12
A13   |   85   DDRCLKOUTP0
D10   |   86   DDRDQS0N
D9   |   87   DDRD07
C10   |   88   DDRDQM0
C20   |   89   DDRD22
C9   |   90   DDRD06
C14   |   91   DDRBA0
A7   |   92   DDRD13
A12   |   93   DDRD00
P25   |   94   AEA16
AD26  |   95   AED12
AF24  |   96   AED03
N26   |   97   AEA07
U25   |   98   AEA00
V25   |   99   ABA0
F27   |   100   AED52
T25   |   101   AEA11
G26   |   102   AED50
AB25  |   103   AED26
H26   |   104   AED43
Y27   |   105   AED27
AC24  |   106   AED00
C28   |   107   AED41
J24   |   108   AED47
R26   |   109   AEA13
G27   |   110   AED48
AF28  |   111   AED30
B27   |   112   AED51
W27   |   113   ABE02Z
D25   |   114   AED57
D28   |   115   AED39
K25   |   116   AED46
AA24  |   117   ASDWEZ
L24   |   118   AED33
AE28  |   119   AED19
U28   |   120   AEA05
AE25  |   121   AOE
AG25  |   122   AED14
AB26  |   123   AED28
AA27  |   124   AED22
AF25  |   125   AED09
V26   |   126   ACE5Z
G25   |   127   AED36
R25   |   128   AADS
Y24   |   129   ABE01Z
AA25  |   130   AED23
T26   |   131   AEA02
N25   |   132   AHOLDAZ
J25   |   133   AED45
AC25  |   134   AED11
AB24  |   135   AED24
M26   |   136   AEA09
Y28   |   137   ABE03Z
G28   |   138   AED35
AE24  |   139   AED01
K28   |   140   AARDY
L28   |   141   ABE05Z
M24   |   142   AEA17
AC26  |   143   AED08
D27   |   144   AED58
W26   |   145   ACE2Z
AA28  |   146   AED29
N24   |   147   AEA10
E26   |   148   AED59
AE27  |   149   AED15
AF27  |   150   AED18
V24   |   151   ABA1
B26   |   152   AED49
C26   |   153   AED61
T28   |   154   AEA06
H24   |   155   AED55
AG27  |   156   AED20
U27   |   157   ACE4Z
J28   |   158   AED40
AC27  |   159   AED13
W28   |   160   ABE07Z
D26   |   161   AED53
T27   |   162   AEA03
AD27  |   163   AED04
AH26  |   164   AED06
N28   |   165   AECLKIN
Y25   |   166   ABE00Z
J26   |   167   AED44
A26   |   168   AED62
C27   |   169   AED60
H25   |   170   AED54
AF26  |   171   AED16
M25   |   172   AEA18
L27   |   173   ABE04Z
AE26  |   174   AED10
G24   |   175   AED63
K27   |   176   AED34
L26   |   177   ABUSREQ0
K24   |   178   AED38
U26   |   179   AEA01
Y26   |   180   AED31
W25   |   181   ACE3Z
P24   |   182   AEA19
AD28  |   183   AED17
F26   |   184   AED56
W24   |   185   ARNW
T24   |   186   AEA14
R24   |   187   AEA08
R27   |   188   AEA04
F28   |   189   AED37
P26   |   190   AEA15
J27   |   191   AED42
K26   |   192   AED32
N27   |   193   AEA12
AG26  |   194   AED02
AH25  |   195   AED05
AC28  |   196   AED21
V28   |   197   AECLKOUT
L25   |   198   ABE06Z
R28   |   199   AHOLDZ
AA26  |   200   AED25
AD25  |   201   AED07
AE4   |   202   EMU03
AH5   |   203   EMU02
AD5   |   204   EMU00
AD1   |   205   EMU15
AE3   |   206   EMU10
AG4   |   207   EMU05
AF2   |   208   EMU11
Y2   |   209   TMS
AA1   |   210   EMU17
AE1   |   211   EMU12
AG2   |   212   EMU07
AB1   |   213   TDI
AF3   |   214   EMU13
AF4   |   215   EMU06
AC1   |   216   EMU14
AD3   |   217   EMU16
AH3   |   218   TCK
AC2   |   219   EMU18
AE5   |   220   EMU01
AH4   |   221   EMU04
AE2   |   222   TRSTZ
AG3   |   223   EMU08
AF1   |   224   TDO
AD4   |   225   EMU09
D24   |   226   GP12
B25   |   227   GP08
C5   |   228   GP06
B5   |   229   GP04
F5   |   230   GP07
C25   |   231   GP11
B4   |   232   GP03
D5   |   233   GP02
A5   |   234   GP00
E5   |   235   GP01
A25   |   236   GP10
F6   |   237   GP05
C24   |   238   GP09
D23   |   239   GP14
F23   |   240   GP15
C23   |   241   GP13
R1   |   242   HD17
W1   |   243   HD11
P3   |   244   HD31
V1   |   245   HD22
T3   |   246   HD09
L2   |   247   HDS1Z
M1   |   248   HD24
W2   |   249   HD00
L6   |   250   HCNTL0
N4   |   251   HD12
U4   |   252   HD05
R6   |   253   HD04
N3   |   254   HD16
N5   |   255   HD08
R5   |   256   HD10
P4   |   257   HD14
U5   |   258   HD27
M6   |   259   HRDYZ
N1   |   260   HD26
K5   |   261   HRWZ
L3   |   262   HHWIL
N2   |   263   HD20
U1   |   264   HD21
T1   |   265   HD19
P5   |   266   HD02
T2   |   267   HD15
M3   |   268   HCSZ
N6   |   269   HD30
T5   |   270   HD29
M5   |   271   HCNTL1
U6   |   272   HD23
K6   |   273   HD01
L4   |   274   HINTZ
P2   |   275   HD18
T4   |   276   HD03
R4   |   277   HD07
P6   |   278   HD28
U2   |   279   HD13
L5   |   280   HDS2Z
M4   |   281   HASZ
T6   |   282   HD06
V2   |   283   HD25
F24   |   284   SCL
E24   |   285   SDA
Y6   |   286   DR0
AA4   |   287   CLKS0
V4   |   288   FSR0
W4   |   289   FSX0
Y5   |   290   CLKR0
AB3   |   291   CLKX0
W6   |   292   DX0
AA3   |   293   CLKX1
Y3   |   294   DX1
W3   |   295   DR1
V5   |   296   FSR1
Y1   |   297   CLKS1
W5   |   298   FSX1
Y4   |   299   CLKR1
AH19  |   300   MDIO
AH18  |   301   MDCLK
AF22  |   302   RSV27
AE23  |   303   RSV22
AH22  |   304   RSV29
AG23  |   305   RSV28
AE22  |   306   RSV26
AG19  |   307   TINP1L
AF19  |   308   TOUT1L
AG20  |   309   TOUT0L
AH20  |   310   TINP0L
H3   |   311   UXDATA3
H2   |   312   URADDR0
K1   |   313   URADDR4
J5   |   314   UXADDR1
J1   |   315   URADDR2
F2   |   316   URDATA6
K2   |   317   URADDR3
H5   |   318   UXADDR3
G3   |   319   UXDATA2
C4   |   320   UXDATA5
F1   |   321   URDATA5
E1   |   322   URDATA3
C3   |   323   UXCLAV
C1   |   324   URCLK
K3   |   325   UXADDR2
F3   |   326   UXDATA7
E3   |   327   UXDATA0
B3   |   328   UXENBZ
G2   |   329   URSOC
E4   |   330   UXDATA6
A3   |   331   UXDATA4
D2   |   332   URDATA2
D1   |   333   URDATA1
A4   |   334   UXCLK
G4   |   335   UXSOC
C2   |   336   URDATA0
E2   |   337   URDATA4
K4   |   338   URENBZ
H4   |   339   UXADDR0
J3   |   340   URADDR1
G1   |   341   URDATA7
F4   |   342   UXDATA1
B2   |   343   URCLAV
J4   |   344   UXADDR4
[Model Data]
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[End Model Data]
[End Package Model]
| Models and submodels in the file (56): BC1840DTHYPDFZ (I/O), BC1840ETHYFZ (I/O), ICLKRX18G (Input), IC18THYPUFZ (Input), IC18THYPDFZ (Input), IC18THY (Input), IC18GHY (Input), BI2C18TFZ (I/O_open_drain), BC1850CTHYPUFZ (I/O), BC1840ETHYPDFZ (I/O), BC1825ETHYPUFZ (I/O), BC1825ETHYPDFZ (I/O), BQ3350ZTCBTHYPBFZP18 (I/O), BQ3340ZTCDTHYPBFZP18 (I/O), NOSR0_10PER_45OHM_1P8 (3-state), SR0_10PER_45OHM_1P8 (3-state), NOSR0_5PER_45OHM_1P8 (3-state), SR0_5PER_45OHM_1P8 (3-state), NOSR0_10PER_50OHM_1P8 (3-state), SR0_10PER_50OHM_1P8 (3-state), NOSR0_5PER_50OHM_1P8 (3-state), SR0_5PER_50OHM_1P8 (3-state), NOSR0_10PER_55OHM_1P8 (3-state), SR0_10PER_55OHM_1P8 (3-state), NOSR0_5PER_55OHM_1P8 (3-state), SR0_5PER_55OHM_1P8 (3-state), NOSR0_10PER_30OHM_1P8 (3-state), SR0_10PER_30OHM_1P8 (3-state), NOSR0_5PER_30OHM_1P8 (3-state), SR0_5PER_30OHM_1P8 (3-state), 45OHM_10PER_HALFTERM_1P8 (Input), 45OHM_10PER_NOTERM_1P8 (Input), 45OHM_10PER_FULLTERM_1P8 (Input), 45OHM_5PER_HALFTERM_1P8 (Input), 45OHM_5PER_NOTERM_1P8 (Input), 45OHM_5PER_FULLTERM_1P8 (Input), 50OHM_10PER_HALFTERM_1P8 (Input), 50OHM_10PER_NOTERM_1P8 (Input), 50OHM_10PER_FULLTERM_1P8 (Input), 50OHM_5PER_HALFTERM_1P8 (Input), 50OHM_5PER_NOTERM_1P8 (Input), 50OHM_5PER_FULLTERM_1P8 (Input), 55OHM_10PER_HALFTERM_1P8 (Input), 55OHM_10PER_NOTERM_1P8 (Input), 55OHM_10PER_FULLTERM_1P8 (Input), 55OHM_5PER_HALFTERM_1P8 (Input), 55OHM_5PER_NOTERM_1P8 (Input), 55OHM_5PER_FULLTERM_1P8 (Input), 30OHM_10PER_HALFTERM_1P8 (Input), 30OHM_10PER_NOTERM_1P8 (Input), 30OHM_10PER_FULLTERM_1P8 (Input), 30OHM_5PER_HALFTERM_1P8 (Input), 30OHM_5PER_NOTERM_1P8 (Input), 30OHM_5PER_FULLTERM_1P8 (Input), BC1850CTHYPDFZ_PD_1P8 (I/O), BC1850CTHYPDFZ_PDZ_1P8 (I/O)
